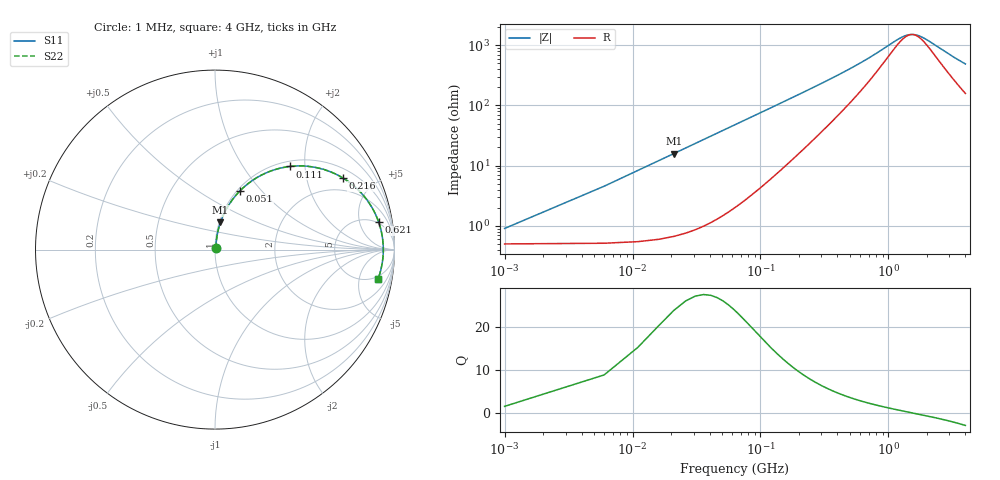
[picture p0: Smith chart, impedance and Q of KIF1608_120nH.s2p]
# MHz S RI R 50
!Freq ReS11 ImS11 ReS21 ImS21 ReS12 ImS12 ReS22 ImS22
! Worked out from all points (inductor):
!   801 points, 1 MHz to 4 GHz, reference 50 ohm
!   read as one part in series: L = 120 nH near 21 MHz
!   highest Q = 23.7 at 21 MHz (marker M1), where L = 120 nH
!   self-resonance near 1.53 GHz
!   S11 on the Smith chart (normalised r, x): 1 MHz: 1.01, +0.02; 51 MHz: 1.03, +0.77; 111 MHz: 1.10, +1.68; 216 MHz: 1.37, +3.28; 621 MHz: 5, +10; 4 GHz: 4, -9
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1  0.00503 0.00746  0.995 -0.00746  0.995 -0.00746  0.00503 0.00746
11  0.0121 0.0814  0.9879 -0.0814  0.9879 -0.0814  0.0121 0.0814
21  0.0305 0.1523  0.9695 -0.1523  0.9695 -0.1523  0.0305 0.1523
26  0.0436 0.1859  0.9564 -0.1859  0.9564 -0.1859  0.0436 0.1859
31  0.059 0.2178  0.941 -0.2178  0.941 -0.2178  0.059 0.2178
41  0.0956 0.2762  0.9044 -0.2762  0.9044 -0.2762  0.0956 0.2762
51  0.1381 0.3263  0.8619 -0.3263  0.8619 -0.3263  0.1381 0.3263
76  0.2573 0.4144  0.7427 -0.4144  0.7427 -0.4144  0.2573 0.4144
111  0.4182 0.4634  0.5818 -0.4634  0.5818 -0.4634  0.4182 0.4634
161  0.5914 0.4507  0.4086 -0.4507  0.4086 -0.4507  0.5914 0.4507
216  0.7104 0.4005  0.2896 -0.4005  0.2896 -0.4005  0.7104 0.4005
281  0.7921 0.3386  0.2079 -0.3386  0.2079 -0.3386  0.7921 0.3386
361  0.8475 0.2757  0.1525 -0.2757  0.1525 -0.2757  0.8475 0.2757
621  0.9121 0.1526  0.0879 -0.1526  0.0879 -0.1526  0.9121 0.1526
671  0.9171 0.1373  0.0829 -0.1373  0.0829 -0.1373  0.9171 0.1373
1041  0.9339 0.0599  0.0661 -0.0599  0.0661 -0.0599  0.9339 0.0599
1336  0.9373 0.0207  0.0627 -0.0207  0.0627 -0.0207  0.9373 0.0207
1611  0.9378 -0.00792  0.0622 0.00792  0.0622 0.00792  0.9378 -0.00792
2001  0.936 -0.0414  0.064 0.0414  0.064 0.0414  0.936 -0.0414
2671  0.9294 -0.0888  0.0706 0.0888  0.0706 0.0888  0.9294 -0.0888
3336  0.9198 -0.1289  0.0802 0.1289  0.0802 0.1289  0.9198 -0.1289
4000  0.9079 -0.1649  0.0921 0.1649  0.0921 0.1649  0.9079 -0.1649
